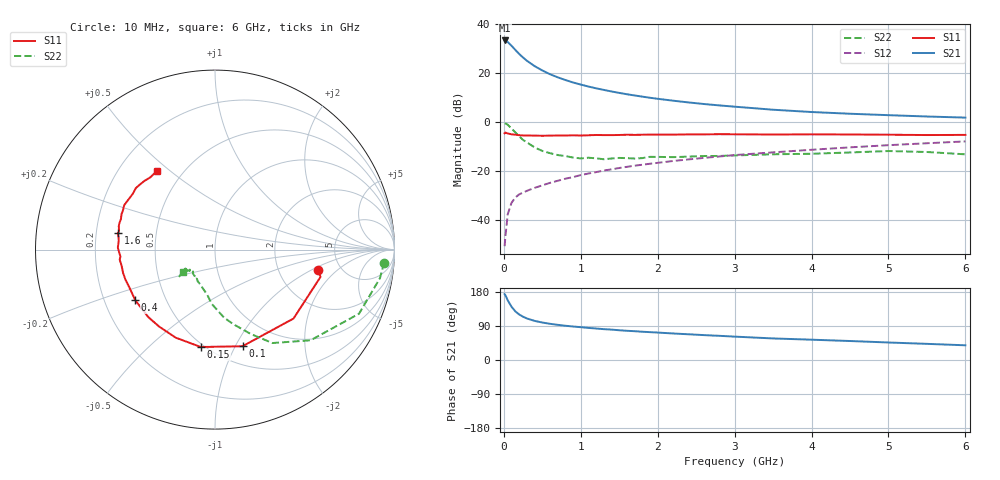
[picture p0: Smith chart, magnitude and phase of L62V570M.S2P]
!  INFINEON TECHNOLOGIES Small Signal Semiconductors
! BFR380L3 , Si-NPN RF-Transistor in TSLP-3-1
!  Vce=2.5 V,  Ic=70 mA
! Common Emitter S-Parameters:  07. March 2005
#  GHz  S  MA  R  50
! f  S11  S21  S12  S22
! GHz  Mag  Ang  Mag  Ang  Mag  Ang  Mag  Ang
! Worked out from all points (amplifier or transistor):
!   36 points, 10 MHz to 6 GHz, reference 50 ohm
!   highest |S21| = 33.3 dB at 10 MHz (marker M1)
!   |S21| within 3 dB of that: start of sweep to 124.3 MHz
!   unconditionally stable (mu >= 1): 1.246 GHz to 4.875 GHz
!   at 250 MHz: K = 0.54, MSG = 27.6 dB, |S12| = -28.9 dB
!   at 1.4 GHz: K = 1.01, MAG = 15.2 dB, |S12| = -19.4 dB
!   at 6 GHz: K = 0.98, MSG = 4.9 dB, |S12| = -7.9 dB
!   S11 on the Smith chart (normalised r, x): 10 MHz: 3.39, -1.20; 100 MHz: 0.68, -1.07; 150 MHz: 0.48, -0.74; 400 MHz: 0.33, -0.26; 1.6 GHz: 0.29, +0.08; 6 GHz: 0.36, +0.45
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0.01  0.5876 -11.4  46.24 173.8  0.0029 82.7  0.9454 -4.4
0.02  0.6073 -14.5  45.92 171.1  0.0045 83.2  0.9328 -9.8
0.05  0.5821 -41.3  42.99 157.7  0.0129 73.5  0.8784 -24.0
0.1  0.5598 -74.1  36.05 140.5  0.0223 63.9  0.734 -43.5
0.15  0.5485 -98.3  29.57 128.2  0.0287 56.8  0.6113 -58.4
0.2  0.5373 -114.1  24.46 120.0  0.0332 54.9  0.5099 -67.1
0.25  0.5298 -126.1  20.72 114.2  0.036 52.8  0.4285 -76.1
0.3  0.5288 -134.7  17.77 109.6  0.0392 53.8  0.3825 -82.4
0.4  0.5264 -147.6  13.83 103.2  0.045 54.9  0.3023 -93.6
0.5  0.5214 -155.9  11.28 98.9  0.0507 57.3  0.2557 -99.6
0.6  0.5262 -161.6  9.444 95.5  0.057 59.4  0.2304 -106.2
0.7  0.5285 -165.8  8.174 92.8  0.0628 61.0  0.2109 -112.7
0.9  0.534 -174.0  6.401 88.4  0.0747 63.9  0.1875 -122.9
1.1  0.5347 -178.5  5.292 84.7  0.0885 65.3  0.186 -127.9
1.3  0.5391 176.2  4.512 81.4  0.1019 66.2  0.173 -135.2
1.6  0.5486 170.5  3.682 77.1  0.1211 66.9  0.1823 -141.4
2.2  0.5512 161.9  2.721 70.0  0.1595 67.3  0.1911 -142.1
2.8  0.5631 153.9  2.179 63.8  0.197 66.8  0.2021 -147.1
3.5  0.5534 145.7  1.778 56.9  0.2393 64.5  0.2187 -145.0
4.5  0.5545 139.6  1.472 50.1  0.3028 62.4  0.2381 -143.7
5.5  0.5401 131.6  1.293 42.6  0.3674 58.3  0.2434 -143.3
6  0.5441 126.7  1.227 38.8  0.4006 56.1  0.2181 -145.9
